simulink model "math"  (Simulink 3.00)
settings: Solver=ode45  StartTime=0.0  StopTime=10.0  RelTol=1e-3
libraries: simulink3 x1

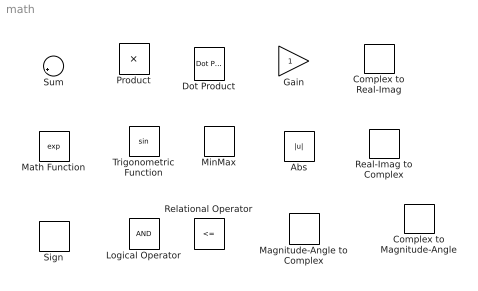
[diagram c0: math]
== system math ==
  Abs : Abs
  Complex to Magnitude-Angle : ComplexToMagnitudeAngle  Output=MagnitudeAndAngle
  Complex to Real-Imag : ComplexToRealImag  Output=RealAndImag
  Dot Product : simulink3/Math/Dot Product
  Gain : Gain  Gain=1  SaturateOnIntegerOverflow=on
  Logical Operator : Logic  Operator=AND  Inputs=2
  Magnitude-Angle to Complex : MagnitudeAngleToComplex  Input=MagnitudeAndAngle  ConstantPart=0
  Math Function : Math  Operator=exp  OutputSignalType=auto
  MinMax : MinMax  Function=min  Inputs=1
  Product : Product  Inputs=2  SaturateOnIntegerOverflow=on
  Real-Imag to Complex : RealImagToComplex  Input=RealAndImag  ConstantPart=0
  Relational Operator : RelationalOperator  Operator=<=
  Sign : Signum
  Sum : Sum  Inputs=|++  SaturateOnIntegerOverflow=on
  Trigonometric Function : Trigonometry  Operator=sin  OutputSignalType=auto
